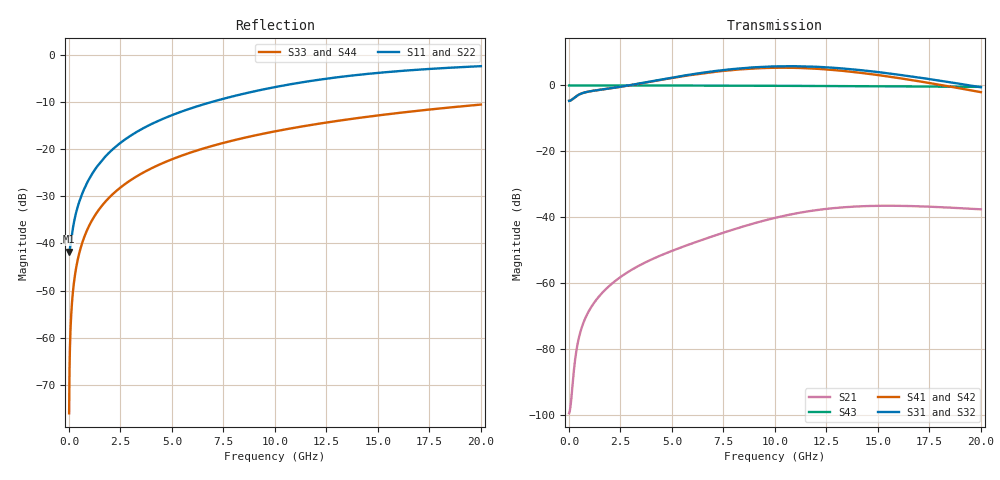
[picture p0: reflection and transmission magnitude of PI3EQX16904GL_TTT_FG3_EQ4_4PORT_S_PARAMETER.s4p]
! NPort=4 DATA=2000 NOISE=0 GROUPDELAY=0 COMPLEX_DATAFORMAT=POLAR
! NumOfBlock=1 NumOfParam=0
! .MODEL Smodel S TSTONEFILE=PI3EQX16904GL_TTT_FG3_EQ4_4PORT_S_PARAMETER.s4p TYPE=S
!  -- The above .MODEL line can be used for the S element in the netlist.
! The s parameter is extracted from the linear redriver, it is not bi-directional; only s(4,1)s(4,2) and s(3,1)s(3,2)
! should be the insertion loss
!Port definition:
!Port1 = input+
!Port2 = input-
!Port3 = output+
!Port4 = output-
# Hz S MA R  50
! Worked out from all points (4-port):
!   2000 points, 10 MHz to 20 GHz, reference 50 ohm
!   strongest paths, dB at 10 MHz, 5.01 GHz, 10.01 GHz, 15.01 GHz, 20 GHz:
!     S31: -4.7, 2.4, 5.8, 4.1, -0.5
!     S32: -4.7, 2.2, 5.6, 3.9, -0.7
!     S41: -4.7, 2.3, 5.4, 3.1, -2.0
!     S42: -4.7, 2.0, 5.2, 3.0, -2.2
!     S43: 0.0, 0.0, -0.1, -0.3, -0.4
!     S21: -99.6, -50.2, -40.2, -36.6, -37.6
!   lowest |S11| = -41.7 dB at 10 MHz (marker M1), VSWR 1.02, Z = 49.2 - j0.0603 ohm
!   |S11| at or under -10 dB: start of sweep to 6.892 GHz
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1e7  0.008182 -175.7  1.05e-05 7.7  0 0.0  0 0.0
     1.05e-05 7.7  0.008182 -175.7  0 0.0  0 0.0
     0.5835 0.4  0.5835 -179.6  0.0001571 -90.0  1 -0.0
     0.5835 -179.6  0.5835 0.4  1 -0.0  0.0001571 -90.0
3.9e8  0.02299 -119.3  0.0001055 117.7  0 0.0  0 0.0
       0.0001055 117.7  0.02299 -119.3  0 0.0  0 0.0
       0.6969 9.3  0.6962 -170.9  0.006126 -90.4  1 -0.4
       0.6968 -171.4  0.6962 8.4  1 -0.4  0.006126 -90.4
1.62e9  0.07696 -102.8  0.0007101 106.6  0 0.0  0 0.0
        0.0007099 106.6  0.07697 -102.8  0 0.0  0 0.0
        0.8693 0.5  0.8665 180.0  0.02544 -91.5  0.9997 -1.5
        0.8681 177.6  0.8653 -2.9  0.9997 -1.5  0.02544 -91.5
6.04e9  0.2773 -105.1  0.004081 88.1  0 0.0  0 0.0
        0.004054 88.2  0.2773 -105.1  0 0.0  0 0.0
        1.486 -40.6  1.443 138.9  0.09442 -95.6  0.9952 -5.4
        1.459 128.7  1.417 -51.8  0.9952 -5.4  0.09442 -95.6
9.76e9  0.4468 -112.3  0.009418 61.9  0 0.0  0 0.0
        0.009339 62.6  0.4464 -112.4  0 0.0  0 0.0
        1.937 -99.1  1.889 81.0  0.1514 -99.1  0.9875 -8.7
        1.849 63.8  1.803 -116.0  0.9875 -8.7  0.1514 -99.1
1.374e10  0.6071 -122.3  0.01446 17.9  0 0.0  0 0.0
          0.01439 19.0  0.6064 -122.3  0 0.0  0 0.0
          1.758 -167.5  1.722 12.6  0.2106 -102.7  0.9758 -12.2
          1.609 -10.8  1.576 169.4  0.9758 -12.2  0.2106 -102.7
2e10  0.7635 -135.9  0.0132 -35.2  0 0.0  0 0.0
      0.01315 -33.8  0.763 -135.9  0 0.0  0 0.0
      0.9388 102.9  0.9214 -77.0  0.2986 -108.1  0.9506 -17.4
      0.7905 -109.0  0.7758 71.1  0.9506 -17.4  0.2986 -108.1
